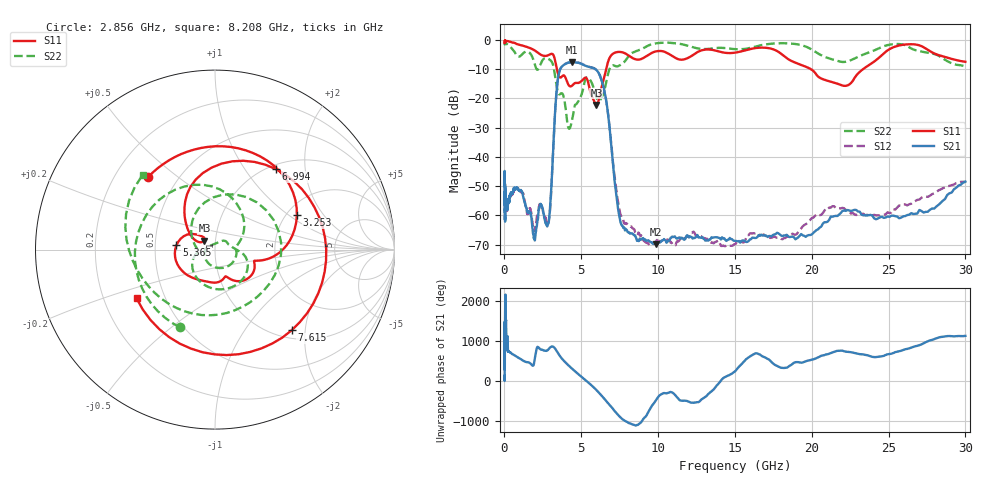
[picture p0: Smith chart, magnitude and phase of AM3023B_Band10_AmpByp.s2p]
# Hz S DB R 50.0
!freq dBS11 angS11 dBS21 angS21 dBS12 angS12 dBS22 angS22
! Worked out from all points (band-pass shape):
!   1601 points, 10 MHz to 30 GHz, reference 50 ohm
!   highest |S21| = -7.63 dB at 4.37 GHz (marker M1); lowest = -69.9 dB at 9.878 GHz (marker M2)
!   |S21| within 3 dB of the highest: 3.585 GHz to 6.048 GHz (2.463 GHz wide, 51.1 % of centre)
!   lowest |S11| = -22.2 dB at 5.989 GHz (marker M3), VSWR 1.17, Z = 44.2 + j4.43 ohm
!   |S11| at or under -10 dB: 3.412 GHz to 6.62 GHz (3.208 GHz wide, 63.9 % of centre); 19.94 GHz to 23.34 GHz (3.395 GHz wide, 15.7 % of centre)
!   |S22| runs from -30.4 to -0.8 dB; largest |S21 - S12| = 0.0097
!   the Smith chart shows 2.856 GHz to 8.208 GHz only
!   S11 on the Smith chart (normalised r, x): 2.856 GHz: 0.34, +0.39; 3.253 GHz: 2.27, +1.15; 5.365 GHz: 0.64, +0.03; 6.994 GHz: 1.07, +1.40; 7.615 GHz: 1.16, -1.69; 8.208 GHz: 0.34, -0.25
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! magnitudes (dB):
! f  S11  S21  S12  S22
! 10 MHz  -0.4  -49.8  -49.4  -0.9
! 38.04 MHz  -0.2  -60.5  -58.9  -0.8
! 54 MHz  -0.4  -51.6  -49.6  -1.2
! 144.7 MHz  -0.3  -54.9  -56.1  -1.3
! 547.7 MHz  -0.9  -52.0  -52.4  -3.4
! 1.115 GHz  -1.8  -51.7  -52.1  -5.1
! 2.084 GHz  -4.0  -64.1  -61.6  -9.9
! 2.349 GHz  -5.0  -56.1  -56.2  -8.3
! 2.856 GHz  -5.2  -62.8  -62.2  -6.5
! 3.253 GHz  -6.1  -28.7  -28.6  -10.9
! 3.577 GHz  -12.7  -10.8  -10.7  -18.6
! 4.37 GHz  -15.8  -7.6  -7.6  -28.2
! 5.365 GHz  -13.3  -9.0  -9.0  -12.8
! 5.989 GHz  -22.2  -10.3  -10.3  -19.7
! 6.521 GHz  -12.2  -17.9  -17.9  -16.7
! 6.994 GHz  -5.0  -38.6  -37.8  -8.7
! 7.615 GHz  -4.2  -63.2  -60.6  -8.3
! 7.926 GHz  -4.8  -64.9  -63.0  -6.7
! 8.208 GHz  -5.8  -66.2  -63.8  -4.7
! 9.878 GHz  -3.9  -69.9  -69.0  -1.1
! 19.31 GHz  -8.6  -66.4  -64.4  -1.8
! 30 GHz  -7.5  -48.5  -48.5  -9.1
